| / 7\'7   Xilinx XC17S00 I/O Buffer IBIS File
| \ \   Xilinx Inc.
| / /   2100 Logic Drive
| \_\/.\   San Jose,   CA 95124
[IBIS ver]   2.1
[File name]   xc17s00.ibs
[File Rev]   1.0
[Date]   Feb. 07, 2000
[Source]   Spice netlist
[Notes]   - Best/worse process data included in the model
   - Created by Joey Jia x4437
[Disclaimer] The data in this model is derived from SPICE simulations
   using modeling information extracted from the target pro-
   cess. While a great deal of care has been take to provide
   information that is accurate, this model is considered
   preliminary as it has not been verified by actual silicon
   measurement. Treat the data in this model as preliminary
   until actual silicon verification is performed.
[Copyright]   Xilinx Inc. All right reserved
|   Component XC17S05_PD8
[Component]   XC17S05_PD8
[Manufacturer]   Xilinx Inc.
[Package]
| variable   typ   min   max
R_pkg   89.00m   80.000m   98.00m
L_pkg   5.850nH   4.200nH   7.500nH
C_pkg   0.950pF   0.700pF   1.200pF
[Pin]  signal_name   model_name   R_pin   L_pin   C_pin
io   datap   IO_S00   NA   NA   NA
| End [Component] XC17S05_PD8
|   Component XC17S05_VO8
[Component]   XC17S05_VO8
[Manufacturer]   Xilinx Inc.
[Package]
| variable   typ   min   max
R_pkg   42.50m   41.000m   44.00m
L_pkg   1.800nH   1.600nH   2.000nH
C_pkg   0.300pF   0.300pF   0.300pF
[Pin]  signal_name   model_name   R_pin   L_pin   C_pin
io   datap   IO_S00   NA   NA   NA
| End [Component] XC17S05_VO8
|   Component XC17S10_PD8
[Component]   XC17S10_PD8
[Manufacturer]   Xilinx Inc.
[Package]
| variable   typ   min   max
R_pkg   89.00m   80.000m   98.00m
L_pkg   5.850nH   4.200nH   7.500nH
C_pkg   0.950pF   0.700pF   1.200pF
[Pin]  signal_name   model_name   R_pin   L_pin   C_pin
io   datap   IO_S00   NA   NA   NA
| End [Component] XC17S10_PD8
|   Component XC17S10_VO8
[Component]   XC17S10_VO8
[Manufacturer]   Xilinx Inc.
[Package]
| variable   typ   min   max
R_pkg   42.50m   41.000m   44.00m
L_pkg   1.800nH   1.600nH   2.000nH
C_pkg   0.300pF   0.300pF   0.300pF
[Pin]  signal_name   model_name   R_pin   L_pin   C_pin
io   datap   IO_S00   NA   NA   NA
| End [Component] XC17S10_VO8
|   Component XC17S20_PD8
[Component]   XC17S20_PD8
[Manufacturer]   Xilinx Inc.
[Package]
| variable   typ   min   max
R_pkg   89.00m   80.000m   98.00m
L_pkg   5.850nH   4.200nH   7.500nH
C_pkg   0.950pF   0.700pF   1.200pF
[Pin]  signal_name   model_name   R_pin   L_pin   C_pin
io   datap   IO_S00   NA   NA   NA
| End [Component] XC17S20_PD8
|   Component XC17S20_VO8
[Component]   XC17S20_VO8
[Manufacturer]   Xilinx Inc.
[Package]
| variable   typ   min   max
R_pkg   42.50m   41.000m   44.00m
L_pkg   1.800nH   1.600nH   2.000nH
C_pkg   0.300pF   0.300pF   0.300pF
[Pin]  signal_name   model_name   R_pin   L_pin   C_pin
io   datap   IO_S00   NA   NA   NA
| End [Component] XC17S20_VO8
|   Component XC17S30_PD8
[Component]   XC17S30_PD8
[Manufacturer]   Xilinx Inc.
[Package]
| variable   typ   min   max
R_pkg   89.00m   80.000m   98.00m
L_pkg   5.850nH   4.200nH   7.500nH
C_pkg   0.950pF   0.700pF   1.200pF
[Pin]  signal_name   model_name   R_pin   L_pin   C_pin
io   datap   IO_S00   NA   NA   NA
| End [Component] XC17S30_PD8
|   Component XC17S30_VO8
[Component]   XC17S30_VO8
[Manufacturer]   Xilinx Inc.
[Package]
| variable   typ   min   max
R_pkg   42.50m   41.000m   44.00m
L_pkg   1.800nH   1.600nH   2.000nH
C_pkg   0.300pF   0.300pF   0.300pF
[Pin]  signal_name   model_name   R_pin   L_pin   C_pin
io   datap   IO_S00   NA   NA   NA
| End [Component] XC17S30_VO8
|   Component XC17S40_PD8
[Component]   XC17S40_PD8
[Manufacturer]   Xilinx Inc.
[Package]
| variable   typ   min   max
R_pkg   89.00m   80.000m   98.00m
L_pkg   5.840nH   4.160nH   7.520nH
C_pkg   0.935pF   0.720pF   1.150pF
[Pin]  signal_name   model_name   R_pin   L_pin   C_pin
io   datap   IO_S01   NA   NA   NA
| End [Component] XC17S40_PD8
|   Component XC17S40_SO20
[Component]   XC17S40_SO20
[Manufacturer]   Xilinx Inc.
[Package]
| variable   typ   min   max
R_pkg   51.50m   44.000m   59.00m
L_pkg   3.155nH   1.960nH   4.350nH
C_pkg   0.585pF   0.350pF   0.820pF
[Pin]  signal_name   model_name   R_pin   L_pin   C_pin
io   datap   IO_S01   NA   NA   NA
| End [Component] XC17S40_SO20
|   Component XC17S05XL_PD8
[Component]   XC17S05XL_PD8
[Manufacturer]   Xilinx Inc.
[Package]
| variable   typ   min   max
R_pkg   89.00m   80.000m   98.00m
L_pkg   5.850nH   4.200nH   7.500nH
C_pkg   0.950pF   0.700pF   1.200pF
[Pin]  signal_name   model_name   R_pin   L_pin   C_pin
io   datap   IO_S00L   NA   NA   NA
| End [Component] XC17S05XL_PD8
|   Component XC17S05XL_VO8
[Component]   XC17S05XL_VO8
[Manufacturer]   Xilinx Inc.
[Package]
| variable   typ   min   max
R_pkg   42.50m   41.000m   44.00m
L_pkg   1.800nH   1.600nH   2.000nH
C_pkg   0.300pF   0.300pF   0.300pF
[Pin]  signal_name   model_name   R_pin   L_pin   C_pin
io   datap   IO_S00L   NA   NA   NA
| End [Component] XC17S05XL_VO8
|   Component XC17S10XL_PD8
[Component]   XC17S10XL_PD8
[Manufacturer]   Xilinx Inc.
[Package]
| variable   typ   min   max
R_pkg   89.00m   80.000m   98.00m
L_pkg   5.850nH   4.200nH   7.500nH
C_pkg   0.950pF   0.700pF   1.200pF
[Pin]  signal_name   model_name   R_pin   L_pin   C_pin
io   datap   IO_S00L   NA   NA   NA
| End [Component] XC17S10XL_PD8
|   Component XC17S10XL_VO8
[Component]   XC17S10XL_VO8
[Manufacturer]   Xilinx Inc.
[Package]
| variable   typ   min   max
R_pkg   42.50m   41.000m   44.00m
L_pkg   1.800nH   1.600nH   2.000nH
C_pkg   0.300pF   0.300pF   0.300pF
[Pin]  signal_name   model_name   R_pin   L_pin   C_pin
io   datap   IO_S00L   NA   NA   NA
| End [Component] XC17S10XL_VO8
|   Component XC17S15XL_PD8
[Component]   XC17S15XL_PD8
[Manufacturer]   Xilinx Inc.
[Package]
| variable   typ   min   max
R_pkg   89.00m   80.000m   98.00m
L_pkg   5.850nH   4.200nH   7.500nH
C_pkg   0.950pF   0.700pF   1.200pF
[Pin]  signal_name   model_name   R_pin   L_pin   C_pin
io   datap   IO_S00L   NA   NA   NA
| End [Component] XC17S15XL_PD8
|   Component XC17S15XL_VO8
[Component]   XC17S15XL_VO8
[Manufacturer]   Xilinx Inc.
[Package]
| variable   typ   min   max
R_pkg   42.50m   41.000m   44.00m
L_pkg   1.800nH   1.600nH   2.000nH
C_pkg   0.300pF   0.300pF   0.300pF
[Pin]  signal_name   model_name   R_pin   L_pin   C_pin
io   datap   IO_S00L   NA   NA   NA
| End [Component] XC17S15XL_VO8
|   Component XC17S20XL_PD8
[Component]   XC17S20XL_PD8
[Manufacturer]   Xilinx Inc.
[Package]
| variable   typ   min   max
R_pkg   89.00m   80.000m   98.00m
L_pkg   5.850nH   4.200nH   7.500nH
C_pkg   0.950pF   0.700pF   1.200pF
[Pin]  signal_name   model_name   R_pin   L_pin   C_pin
io   datap   IO_S00L   NA   NA   NA
| End [Component] XC17S20XL_PD8
|   Component XC17S20XL_VO8
[Component]   XC17S20XL_VO8
[Manufacturer]   Xilinx Inc.
[Package]
| variable   typ   min   max
R_pkg   42.50m   41.000m   44.00m
L_pkg   1.800nH   1.600nH   2.000nH
C_pkg   0.300pF   0.300pF   0.300pF
[Pin]  signal_name   model_name   R_pin   L_pin   C_pin
io   datap   IO_S00L   NA   NA   NA
| End [Component] XC17S20XL_VO8
|   Component XC17S30XL_PD8
[Component]   XC17S30XL_PD8
[Manufacturer]   Xilinx Inc.
[Package]
| variable   typ   min   max
R_pkg   89.00m   80.000m   98.00m
L_pkg   5.850nH   4.200nH   7.500nH
C_pkg   0.950pF   0.700pF   1.200pF
[Pin]  signal_name   model_name   R_pin   L_pin   C_pin
io   datap   IO_S00L   NA   NA   NA
| End [Component] XC17S30XL_PD8
|   Component XC17S30XL_VO8
[Component]   XC17S30XL_VO8
[Manufacturer]   Xilinx Inc.
[Package]
| variable   typ   min   max
R_pkg   42.50m   41.000m   44.00m
L_pkg   1.800nH   1.600nH   2.000nH
C_pkg   0.300pF   0.300pF   0.300pF
[Pin]  signal_name   model_name   R_pin   L_pin   C_pin
io   datap   IO_S00L   NA   NA   NA
| End [Component] XC17S30XL_VO8
|   Component XC17S40XL_PD8
[Component]   XC17S40XL_PD8
[Manufacturer]   Xilinx Inc.
[Package]
| variable   typ   min   max
R_pkg   89.00m   80.000m   98.00m
L_pkg   5.840nH   4.160nH   7.520nH
C_pkg   0.935pF   0.720pF   1.150pF
[Pin]  signal_name   model_name   R_pin   L_pin   C_pin
io   datap   IO_S01L   NA   NA   NA
| End [Component] XC17S40XL_PD8
|   Component XC17S40XL_SO20
[Component]   XC17S40XL_SO20
[Manufacturer]   Xilinx Inc.
[Package]
| variable   typ   min   max
R_pkg   51.50m   44.000m   59.00m
L_pkg   3.155nH   1.960nH   4.350nH
C_pkg   0.585pF   0.350pF   0.820pF
[Pin]  signal_name   model_name   R_pin   L_pin   C_pin
io   datap   IO_S01L   NA   NA   NA
| End [Component] XC17S40XL_SO20
|   Component XC17S50XL_PD8
[Component]   XC17S50XL_PD8
[Manufacturer]   Xilinx Inc.
[Package]
| variable   typ   min   max
R_pkg   89.00m   80.000m   98.00m
L_pkg   5.840nH   4.160nH   7.520nH
C_pkg   0.935pF   0.720pF   1.150pF
[Pin]  signal_name   model_name   R_pin   L_pin   C_pin
io   datap   IO_S01L   NA   NA   NA
| End [Component] XC17S50XL_PD8
|   Component XC17S50XL_SO20
[Component]   XC17S50XL_SO20
[Manufacturer]   Xilinx Inc.
[Package]
| variable   typ   min   max
R_pkg   51.50m   44.000m   59.00m
L_pkg   3.155nH   1.960nH   4.350nH
C_pkg   0.585pF   0.350pF   0.820pF
[Pin]  signal_name   model_name   R_pin   L_pin   C_pin
io   datap   IO_S01L   NA   NA   NA
| End [Component] XC17S50XL_SO20
|   Component XC17S100XL_PD8
[Component]   XC17S100XL_PD8
[Manufacturer]   Xilinx Inc.
[Package]
| variable   typ   min   max
R_pkg   89.00m   80.000m   98.00m
L_pkg   5.840nH   4.160nH   7.520nH
C_pkg   0.935pF   0.720pF   1.150pF
[Pin]  signal_name   model_name   R_pin   L_pin   C_pin
io   datap   IO_S01L   NA   NA   NA
| End [Component] XC17S100XL_PD8
|   Component XC17S100XL_SO20
[Component]   XC17S100XL_SO20
[Manufacturer]   Xilinx Inc.
[Package]
| variable   typ   min   max
R_pkg   51.50m   44.000m   59.00m
L_pkg   3.155nH   1.960nH   4.350nH
C_pkg   0.585pF   0.350pF   0.820pF
[Pin]  signal_name   model_name   R_pin   L_pin   C_pin
io   datap   IO_S01L   NA   NA   NA
| End [Component] XC17S100XL_SO20
|   Component XC17S150XL_PD8
[Component]   XC17S150XL_PD8
[Manufacturer]   Xilinx Inc.
[Package]
| variable   typ   min   max
R_pkg   89.00m   80.000m   98.00m
L_pkg   5.840nH   4.160nH   7.520nH
C_pkg   0.935pF   0.720pF   1.150pF
[Pin]  signal_name   model_name   R_pin   L_pin   C_pin
io   datap   IO_S01L   NA   NA   NA
| End [Component] XC17S150XL_PD8
|   Component XC17S150XL_SO20
[Component]   XC17S150XL_SO20
[Manufacturer]   Xilinx Inc.
[Package]
| variable   typ   min   max
R_pkg   51.50m   44.000m   59.00m
L_pkg   3.155nH   1.960nH   4.350nH
C_pkg   0.585pF   0.350pF   0.820pF
[Pin]  signal_name   model_name   R_pin   L_pin   C_pin
io   datap   IO_S01L   NA   NA   NA
| End [Component] XC17S150XL_SO20
| Models and submodels in the file (4): IO_S00 (I/O), IO_S00L (I/O), IO_S01 (I/O), IO_S01L (I/O)
